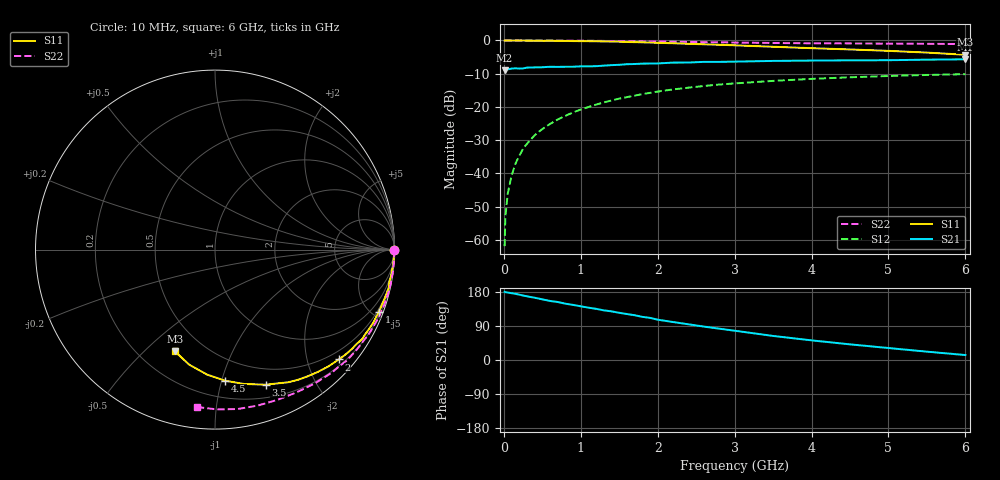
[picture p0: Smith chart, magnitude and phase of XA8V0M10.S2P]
! SIEMENS Discrete & RF Semiconductors
! BFY180
! Si NPN RF Bipolar Junction Transistor in MICRO-X
! VCE = 8 V  IC = 0.1 mA
! Common Emitter S-Parameters:  May  1997
# GHz  S  MA  R  50
!  f  S11  S21  S12  S22
! GHz  MAG  ANG  MAG  ANG  MAG  ANG  MAG  ANG
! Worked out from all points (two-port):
!   36 points, 10 MHz to 6 GHz, reference 50 ohm
!   highest |S21| = -5.68 dB at 6 GHz (marker M1); lowest = -9.0 dB at 10 MHz (marker M2)
!   |S21| within 3 dB of the highest: 17.34 MHz to 49.2 MHz (31.86 MHz wide, 95.8 % of centre); 50.74 MHz to end of sweep
!   lowest |S11| = -4.3 dB at 6 GHz (marker M3), VSWR 4.11, Z = 17.3 - j31.1 ohm
!   |S11| at or under -10 dB: nowhere
!   |S22| runs from -1.1 to 0.0 dB; largest |S21 - S12| = 0.39
!   S11 on the Smith chart (normalised r, x): 10 MHz: open; 1 GHz: 0.36, -5.45; 2 GHz: 0.32, -2.60; 3.5 GHz: 0.33, -1.39; 4.5 GHz: 0.33, -1.03; 6 GHz: 0.35, -0.62
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0.01  0.9968 -0.1  0.355 179.9  0.0008 81.7  0.9999 -0.2
0.02  1 -0.3  0.373 178.9  0.0022 93.1  0.9999 -0.5
0.05  0.9967 -0.9  0.368 178.1  0.0049 84.6  0.9999 -1.0
0.1  0.9972 -2.0  0.377 176.3  0.0092 87.1  0.9985 -1.9
0.15  0.9966 -3.2  0.381 174.6  0.0139 88.0  0.9999 -2.8
0.25  0.9978 -5.4  0.379 170.1  0.0234 86.5  0.9999 -4.6
0.4  0.9922 -8.4  0.393 164.3  0.0373 82.9  0.9989 -7.4
0.5  0.9879 -10.6  0.395 160.1  0.0464 80.6  0.9975 -9.3
0.7  0.9866 -14.6  0.4 153.1  0.0645 76.3  0.9961 -13.1
1  0.9768 -20.7  0.408 141.7  0.0914 70.4  0.9909 -18.7
1.1  0.9731 -22.9  0.407 138.1  0.0995 68.8  0.9884 -20.4
1.5  0.9594 -31.4  0.43 124.6  0.1331 60.8  0.979 -27.8
1.9  0.9299 -39.6  0.449 111.2  0.1624 53.2  0.9667 -35.0
2  0.9221 -41.6  0.451 106.4  0.17 51.5  0.9643 -36.7
2.2  0.9075 -45.7  0.464 100.2  0.1833 47.6  0.9591 -40.3
2.8  0.8611 -57.3  0.476 82.7  0.2169 37.4  0.936 -49.9
3.5  0.8036 -69.5  0.492 63.5  0.2462 26.8  0.9159 -60.4
4  0.7655 -77.9  0.498 51.8  0.2641 19.7  0.9064 -67.5
4.5  0.7323 -85.6  0.502 41.3  0.2788 13.2  0.9011 -74.7
5  0.6974 -93.7  0.504 31.6  0.2919 6.8  0.8971 -81.9
5.5  0.6567 -102.7  0.514 22.0  0.3023 0.2  0.8905 -89.3
6  0.6087 -111.6  0.52 13.1  0.3109 -6.3  0.8828 -96.6
